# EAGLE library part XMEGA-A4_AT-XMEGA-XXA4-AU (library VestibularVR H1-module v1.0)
ATxMega a4 Serie
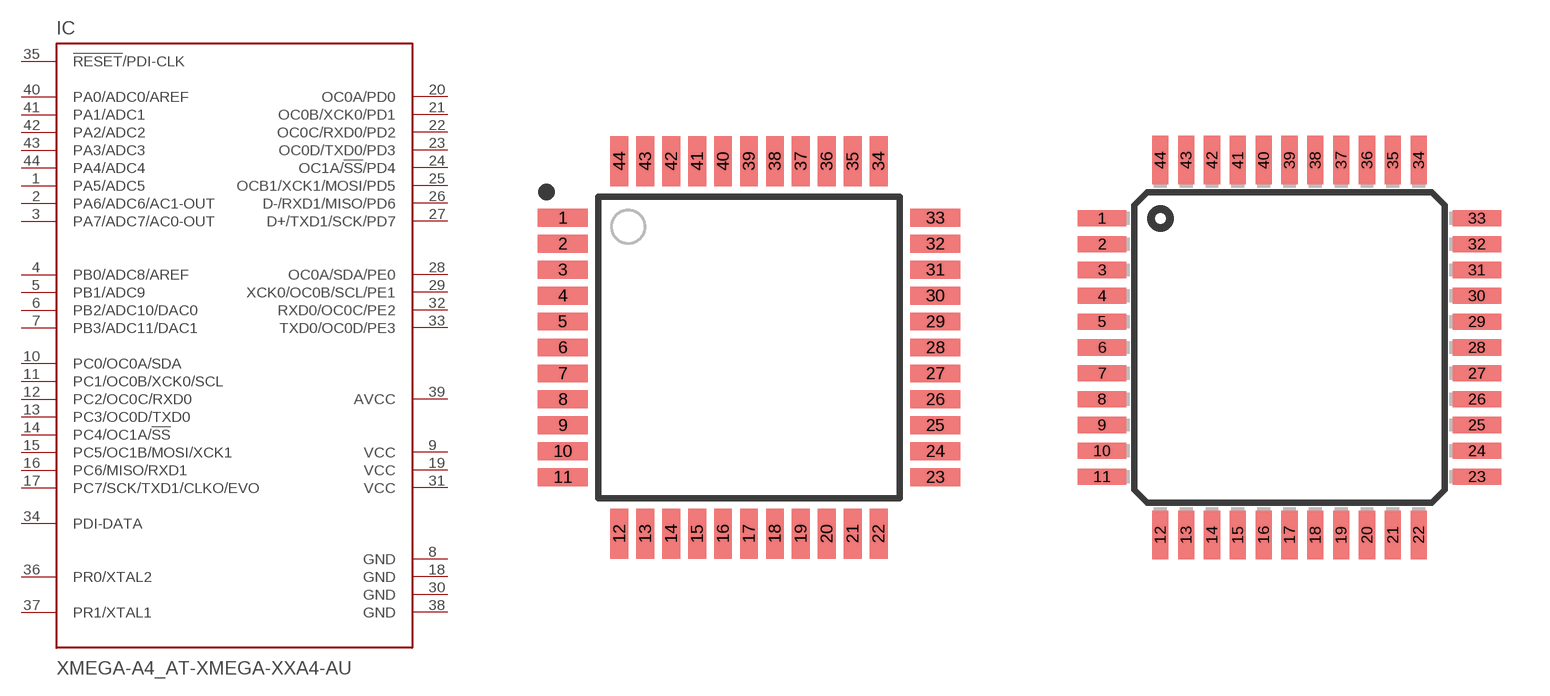
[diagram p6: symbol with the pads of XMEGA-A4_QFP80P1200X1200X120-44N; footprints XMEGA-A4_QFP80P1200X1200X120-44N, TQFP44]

Designator prefix IC

## XMEGA-A4_AT-XMEGA-XXA4-AU  [XMEGA-A4_QFP80P1200X1200X120-44N]
1  PA5/ADC5
2  PA6/ADC6/AC1-OUT
3  PA7/ADC7/AC0-OUT
4  PB0/ADC8/AREF
5  PB1/ADC9
6  PB2/ADC10/DAC0
7  PB3/ADC11/DAC1
8  GND  pwr
9  VCC  pwr
10  PC0/OC0A/SDA
11  PC1/OC0B/XCK0/SCL
12  PC2/OC0C/RXD0
13  PC3/OC0D/TXD0
14  PC4/OC1A/!SS
15  PC5/OC1B/MOSI/XCK1
16  PC6/MISO/RXD1
17  PC7/SCK/TXD1/CLKO/EVO
18  GND  pwr
19  VCC  pwr
20  OC0A/PD0
21  OC0B/XCK0/PD1
22  OC0C/RXD0/PD2
23  OC0D/TXD0/PD3
24  OC1A/!SS!/PD4
25  OCB1/XCK1/MOSI/PD5
26  D-/RXD1/MISO/PD6
27  D+/TXD1/SCK/PD7
28  OC0A/SDA/PE0
29  XCK0/OC0B/SCL/PE1
30  GND  pwr
31  VCC  pwr
32  RXD0/OC0C/PE2
33  TXD0/OC0D/PE3
34  PDI-DATA
35  !RESET!/PDI-CLK  in
36  PR0/XTAL2
37  PR1/XTAL1
38  GND  pwr
39  AVCC  pwr
40  PA0/ADC0/AREF
41  PA1/ADC1
42  PA2/ADC2
43  PA3/ADC3
44  PA4/ADC4

## XMEGA-A4_AT-XMEGA-XXA4-AUTQFP44 (DIGIKEY_PN: ATXMEGA32A4U-AURCT-ND; MOUSER_PN: 556-ATXMEGA32A4U-AU; MPN: ATXMEGA32A4U-AUR)  [TQFP44]
Pads as for XMEGA-A4_QFP80P1200X1200X120-44N

## Footprint XMEGA-A4_QFP80P1200X1200X120-44N (pad centres in mm)
TQFP-44
smd 1.55 x 0.55: 1 -5.75,4; 2 -5.75,3.2; 3 -5.75,2.4; 4 -5.75,1.6; 5 -5.75,0.8; 6 -5.75,0; 7 -5.75,-0.8; 8 -5.75,-1.6; 9 -5.75,-2.4; 10 -5.75,-3.2; 11 -5.75,-4; 23 5.75,-4; 24 5.75,-3.2; 25 5.75,-2.4; 26 5.75,-1.6; 27 5.75,-0.8; 28 5.75,0; 29 5.75,0.8; 30 5.75,1.6; 31 5.75,2.4; 32 5.75,3.2; 33 5.75,4
smd 0.55 x 1.55: 12 -4,-5.75; 13 -3.2,-5.75; 14 -2.4,-5.75; 15 -1.6,-5.75; 16 -0.8,-5.75; 17 0,-5.75; 18 0.8,-5.75; 19 1.6,-5.75; 20 2.4,-5.75; 21 3.2,-5.75; 22 4,-5.75; 34 4,5.75; 35 3.2,5.75; 36 2.4,5.75; 37 1.6,5.75; 38 0.8,5.75; 39 0,5.75; 40 -0.8,5.75; 41 -1.6,5.75; 42 -2.4,5.75; 43 -3.2,5.75; 44 -4,5.75

## Footprint TQFP44 (pad centres in mm)
Thin Quad Flat Pack package type TQ
smd 1.5 x 0.5: 1 -5.8,4; 2 -5.8,3.2; 3 -5.8,2.4; 4 -5.8,1.6; 5 -5.8,0.8; 6 -5.8,0; 7 -5.8,-0.8; 8 -5.8,-1.6; 9 -5.8,-2.4; 10 -5.8,-3.2; 11 -5.8,-4; 23 5.8,-4; 24 5.8,-3.2; 25 5.8,-2.4; 26 5.8,-1.6; 27 5.8,-0.8; 28 5.8,0; 29 5.8,0.8; 30 5.8,1.6; 31 5.8,2.4; 32 5.8,3.2; 33 5.8,4
smd 0.5 x 1.5: 12 -4,-5.8; 13 -3.2,-5.8; 14 -2.4,-5.8; 15 -1.6,-5.8; 16 -0.8,-5.8; 17 0,-5.8; 18 0.8,-5.8; 19 1.6,-5.8; 20 2.4,-5.8; 21 3.2,-5.8; 22 4,-5.8; 34 4,5.8; 35 3.2,5.8; 36 2.4,5.8; 37 1.6,5.8; 38 0.8,5.8; 39 0,5.8; 40 -0.8,5.8; 41 -1.6,5.8; 42 -2.4,5.8; 43 -3.2,5.8; 44 -4,5.8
